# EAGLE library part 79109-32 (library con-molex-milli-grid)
RECEPTACAL
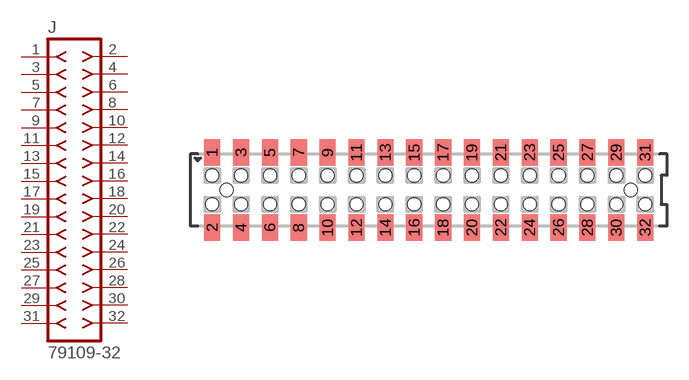
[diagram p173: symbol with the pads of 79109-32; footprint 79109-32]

Designator prefix J

## 79109-32  [79109-32]
1  1  pas
2  2  pas
3  3  pas
4  4  pas
5  5  pas
6  6  pas
7  7  pas
8  8  pas
9  9  pas
10  10  pas
11  11  pas
12  12  pas
13  13  pas
14  14  pas
15  15  pas
16  16  pas
17  17  pas
18  18  pas
19  19  pas
20  20  pas
21  21  pas
22  22  pas
23  23  pas
24  24  pas
25  25  pas
26  26  pas
27  27  pas
28  28  pas
29  29  pas
30  30  pas
31  31  pas
32  32  pas

## Footprint 79109-32 (pad centres in mm)
RECEPTACAL SMD Dual Row, Vertical, Pass-Thru
smd 1.12 x 1.83: 1 -15,2.6; 2 -15,-2.6; 3 -13,2.6; 4 -13,-2.6; 5 -11,2.6; 6 -11,-2.6; 7 -9,2.6; 8 -9,-2.6; 9 -7,2.6; 10 -7,-2.6; 11 -5,2.6; 12 -5,-2.6; 13 -3,2.6; 14 -3,-2.6; 15 -1,2.6; 16 -1,-2.6; 17 1,2.6; 18 1,-2.6; 19 3,2.6; 20 3,-2.6; 21 5,2.6; 22 5,-2.6; 23 7,2.6; 24 7,-2.6; 25 9,2.6; 26 9,-2.6; 27 11,2.6; 28 11,-2.6; 29 13,2.6; 30 13,-2.6; 31 15,2.6; 32 15,-2.6
hole 0.914 at -14,0
hole 0.914 at -15,1
hole 0.914 at -15,-1
hole 0.914 at -13,-1
hole 0.914 at -13,1
hole 0.914 at -11,-1
hole 0.914 at -11,1
hole 0.914 at 14,0
hole 0.914 at -9,1
hole 0.914 at -9,-1
hole 0.914 at -7,1
hole 0.914 at -7,-1
hole 0.914 at -5,1
hole 0.914 at -5,-1
hole 0.914 at -3,1
hole 0.914 at -3,-1
hole 0.914 at -1,-1
hole 0.914 at -1,1
hole 0.914 at 1,1
hole 0.914 at 1,-1
hole 0.914 at 3,1
hole 0.914 at 3,-1
hole 0.914 at 5,1
hole 0.914 at 5,-1
hole 0.914 at 7,-1
hole 0.914 at 7,1
hole 0.914 at 9,1
hole 0.914 at 11,1
hole 0.914 at 13,1
hole 0.914 at 9,-1
hole 0.914 at 11,-1
hole 0.914 at 13,-1
hole 0.914 at 15,-1
hole 0.914 at 15,1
